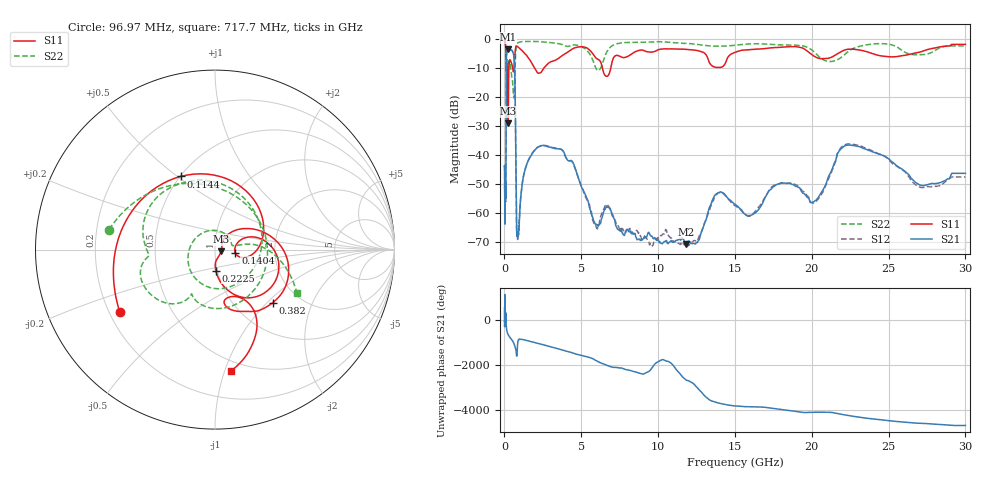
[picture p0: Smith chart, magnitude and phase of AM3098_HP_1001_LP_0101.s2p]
! Date/Time: Thu, Feb 28, 2019 8:40 AM
! Network Analyzer: Agilent Technologies E8364B Rev: A.07.50.67
! Sweep from 0.010 to 30.000 GHz, 1601 Points, Sweep Type: LOG
! Power Supply: 5.023 V, 0.002 A
# Hz S DB R 50
!freq MagS11 AngS11 MagS21 AngS21 MagS12 AngS12 MagS22 AngS22
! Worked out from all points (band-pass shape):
!   1601 points, 10 MHz to 30 GHz, reference 50 ohm
!   highest |S21| = -3.39 dB at 237.5 MHz (marker M1); lowest = -70.9 dB at 11.83 GHz (marker M2)
!   |S21| within 3 dB of the highest: 129.3 MHz to 623 MHz (493.6 MHz wide, 131 % of centre)
!   lowest |S11| = -29.0 dB at 237.5 MHz (marker M3), VSWR 1.07, Z = 53.5 - j1.06 ohm
!   |S11| at or under -10 dB: 199 MHz to 288.1 MHz (89.11 MHz wide, 36.6 % of centre); 1.974 GHz to 2.551 GHz (576.3 MHz wide, 25.5 % of centre); 6.381 GHz to 6.916 GHz (534.5 MHz wide, 8.04 % of centre)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
!   |S22| runs from -20.2 to -0.5 dB; largest |S21 - S12| = 0.012
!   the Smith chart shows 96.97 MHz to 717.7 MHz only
!   S11 on the Smith chart (normalised r, x): 96.97 MHz: 0.24, -0.28; 114.4 MHz: 0.50, +0.51; 140.4 MHz: 1.25, -0.05; 222.5 MHz: 0.98, -0.23; 382 MHz: 1.48, -1.08; 717.7 MHz: 0.41, -1.05
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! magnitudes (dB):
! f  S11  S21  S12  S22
! 10 MHz  -0.3  -43.9  -45.6  -0.5
! 38.04 MHz  -0.5  -61.2  -58.2  -0.8
! 96.97 MHz  -4.0  -44.3  -42.8  -4.4
! 114.4 MHz  -6.9  -16.7  -16.7  -10.6
! 140.4 MHz  -18.8  -4.8  -4.7  -11.1
! 144.7 MHz  -19.0  -4.5  -4.5  -10.6
! 222.5 MHz  -18.6  -3.5  -3.4  -8.5
! 237.5 MHz  -29.0  -3.4  -3.4  -8.7
! 382 MHz  -7.2  -3.7  -3.6  -8.6
! 550.5 MHz  -10.5  -4.4  -4.4  -16.6
! 655.8 MHz  -7.0  -9.2  -9.2  -16.3
! 717.7 MHz  -3.3  -28.7  -28.6  -5.7
! 781.4 MHz  -2.3  -63.0  -63.1  -2.0
! 842.3 MHz  -2.4  -67.8  -68.0  -1.4
! 2.084 GHz  -11.1  -37.6  -37.6  -0.7
! 3.76 GHz  -5.6  -38.2  -38.3  -1.8
! 7.926 GHz  -6.1  -66.0  -66.2  -1.0
! 11.83 GHz  -3.4  -70.9  -71.5  -1.4
! 13.95 GHz  -9.7  -53.0  -53.0  -2.3
! 20.2 GHz  -5.9  -55.8  -56.5  -4.5
! 22.56 GHz  -3.3  -36.6  -36.2  -3.5
! 30 GHz  -1.7  -46.3  -47.6  -2.2
